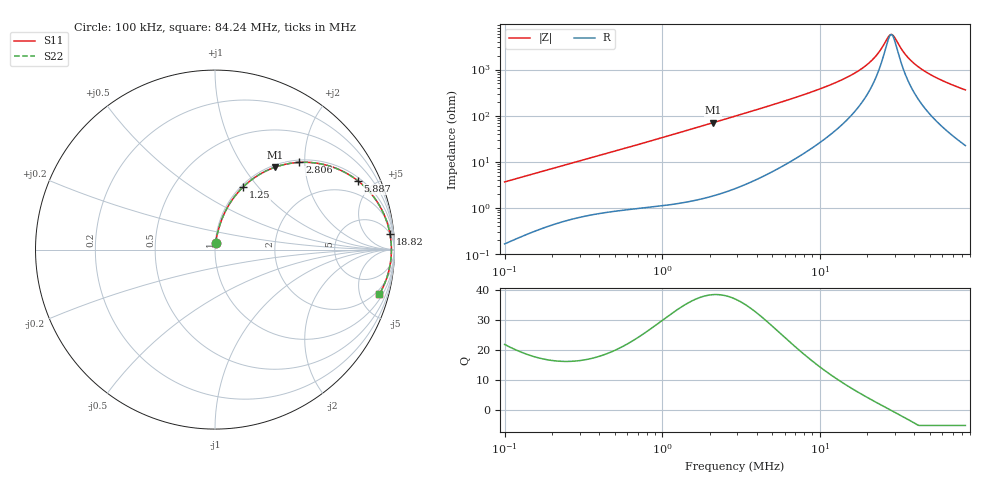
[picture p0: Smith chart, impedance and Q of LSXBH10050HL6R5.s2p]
! LSXBH10050HL6R5  S-PARAMETER MODEL  ( General Type )
! Model Generated by TAIYO YUDEN Corporation (http://www.ty-top.com)
! Version 3.0
! TAIYO YUDEN Control No. 180118NI43SB-FBB
! Copyright(c) 2007 TAIYO YUDEN CO.,LTD. All Rights Reserved.
! Product Description (link to TY-COMPAS)
! https://ds.yuden.co.jp/TYCOMPAS/or/detail?pn=LSXBH10050HL6R5N&u=M
! Products Name : Inductors
! Characteristics :
!  Inductance : 6.5 uH , SRF(min) : 19 MHz , DC Resistance(max) : 0.0234 Ohm
!  Rated Current : Saturation :6000 mA , Temp Rise : 5200 mA (40 degC)
!  Case Size : 10.0 x 9.8 / 0.394 x 0.386 [mm/inch] , Thickness : 5 / 0.197 [mm/inch]
!  (Conditions: Temperature = 25 degC , DC Bias Current/Voltage = 0A / 0V)
! External Node Assignments :
!  1  o---GGG---o  2
! GND o---------o GND
! Frequency Range : 0.1MHz  -  84.23641MHz  [ 402 STEP ]
# MHz S RI R 50
! Freq[MHz].  S11 Real  S11 Imag  S21 Real  S21 Imag  S12 Real  S12 Imag  S22 Real  S22 Imag
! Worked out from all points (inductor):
!   401 points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, 100 kHz to 84.24 MHz, reference 50 ohm
!   read as one part in series: L = 5.78 uH near 103.4 kHz
!   highest Q = 38.6 at 2.108 MHz (marker M1), where L = 5.32 uH
!   self-resonance near 28.19 MHz
!   S11 on the Smith chart (normalised r, x): 100 kHz: 1.00, +0.07; 1.25 MHz: 1.02, +0.84; 2.806 MHz: 1.05, +1.88; 5.887 MHz: 1.16, +4.08; 18.82 MHz: 5, +21; 84.24 MHz: 1.45, -7.20
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0.1  0.003 0.0365  0.997 -0.0365  0.997 -0.0365  0.003 0.0365
0.309045  0.0175 0.1046  0.9825 -0.1046  0.9825 -0.1046  0.0175 0.1046
0.547884  0.0411 0.1762  0.9589 -0.1762  0.9589 -0.1762  0.0411 0.1762
0.955086  0.1007 0.2843  0.8993 -0.2843  0.8993 -0.2843  0.1007 0.2843
1.250439  0.1559 0.3481  0.8441 -0.3481  0.8441 -0.3481  0.1559 0.3481
2.107602  0.3357 0.4595  0.6643 -0.4595  0.6643 -0.4595  0.3357 0.4595
2.806225  0.4706 0.486  0.5294 -0.486  0.5294 -0.486  0.4706 0.486
2.902351  0.4873 0.4866  0.5127 -0.4866  0.5127 -0.4866  0.4873 0.4866
3.996789  0.6427 0.464  0.3573 -0.464  0.3573 -0.464  0.6427 0.464
5.887452  0.7969 0.3826  0.2031 -0.3826  0.2031 -0.3826  0.7969 0.3826
8.96956  0.9024 0.2681  0.0976 -0.2681  0.0976 -0.2681  0.9024 0.2681
13.89724  0.9574 0.1554  0.0426 -0.1554  0.0426 -0.1554  0.9574 0.1554
18.81812  0.9751 0.0865  0.0249 -0.0865  0.0249 -0.0865  0.9751 0.0865
21.17251  0.979 0.0614  0.021 -0.0614  0.021 -0.0614  0.979 0.0614
23.0325  0.9809 0.0438  0.0191 -0.0438  0.0191 -0.0438  0.9809 0.0438
27.71995  0.9829 0.00569  0.0171 -0.00569  0.0171 -0.00569  0.9829 0.00569
28.66948  0.9829 -0.00118  0.0171 0.00118  0.0171 0.00118  0.9829 -0.00118
29.65155  0.9829 -0.00806  0.0171 0.00806  0.0171 0.00806  0.9829 -0.00806
35.68606  0.9808 -0.0462  0.0192 0.0462  0.0192 0.0462  0.9808 -0.0462
43.67809  0.9749 -0.0891  0.0251 0.0891  0.0251 0.0891  0.9749 -0.0891
58.15638  0.9582 -0.1543  0.0418 0.1543  0.0418 0.1543  0.9582 -0.1543
84.23641  0.9154 -0.2488  0.0846 0.2488  0.0846 0.2488  0.9154 -0.2488
